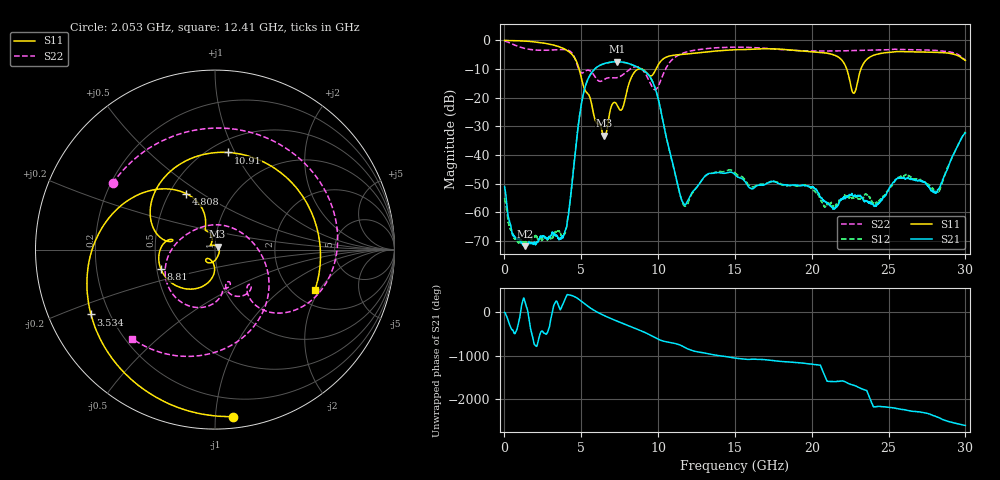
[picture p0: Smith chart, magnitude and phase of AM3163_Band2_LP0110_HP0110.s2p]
!Agilent Technologies,E8364B,MY43040894,A.07.50.67
!Agilent E8364B: A.07.50.67
!Date: Thursday, August 20, 2020 11:12:03
!Correction: S11(Full 2 Port(1,2))
!S21(Full 2 Port(1,2))
!S12(Full 2 Port(1,2))
!S22(Full 2 Port(1,2))
!S2P File: Measurements: S11, S21, S12, S22:
# Hz S  dB  R 50
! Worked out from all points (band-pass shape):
!   3201 points, 10 MHz to 30 GHz, reference 50 ohm
!   highest |S21| = -7.42 dB at 7.348 GHz (marker M1); lowest = -71.7 dB at 1.341 GHz (marker M2)
!   |S21| within 3 dB of the highest: 5.796 GHz to 9.039 GHz (3.244 GHz wide, 43.7 % of centre)
!   lowest |S11| = -33.3 dB at 6.495 GHz (marker M3), VSWR 1.04, Z = 51.4 + j1.67 ohm
!   |S11| at or under -10 dB: 4.86 GHz to 8.714 GHz (3.855 GHz wide, 56.8 % of centre); 8.953 GHz to 9.862 GHz (909.1 MHz wide, 9.66 % of centre); 22.28 GHz to 23.2 GHz (917.5 MHz wide, 4.04 % of centre)
!   |S22| runs from -17.2 to -0.2 dB; largest |S21 - S12| = 0.0047
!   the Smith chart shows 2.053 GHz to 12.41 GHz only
!   S11 on the Smith chart (normalised r, x): 2.053 GHz: 0.07, -1.11; 3.534 GHz: 0.13, -0.24; 4.808 GHz: 0.61, +0.43; 8.81 GHz: 0.53, -0.12; 10.91 GHz: 0.61, +0.94; 12.41 GHz: 2.59, -1.82
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1e7  -0.01 -2.7  -50.94 -9.7  -54.99 -76.7  -0.23 -9.9
6.098e8  -0.08 -24.5  -68.00 -115.6  -69.00 -131.0  -1.50 -81.9
1.340806e9  -0.24 -54.2  -71.75 -133.2  -70.00 -179.4  -2.81 -156.1
2.053069e9  -0.57 -83.9  -70.70 -59.0  -68.19 -64.9  -3.36 147.0
3.533825e9  -2.16 -152.4  -69.25 129.5  -66.59 -24.1  -3.18 43.8
4.05865e9  -3.43 177.1  -64.76 21.8  -64.62 48.4  -3.30 3.1
4.8084e9  -9.08 117.3  -29.48 -60.4  -29.47 -60.9  -9.70 -54.4
5.014581e9  -13.38 106.6  -21.94 -115.8  -21.96 -116.1  -11.34 -47.8
6.495338e9  -33.27 48.3  -8.09 -82.6  -8.10 -82.7  -13.62 -65.8
7.348178e9  -22.69 -133.2  -7.42 148.0  -7.45 147.9  -12.95 -78.6
8.810191e9  -9.89 -160.6  -9.70 -58.4  -9.71 -58.3  -9.51 -139.6
1.000979e10  -8.49 158.6  -20.46 97.2  -20.37 96.6  -15.94 45.9
1.090949e10  -5.25 82.2  -41.99 13.5  -42.20 11.7  -6.73 -58.3
1.167798e10  -4.82 24.6  -56.97 -80.0  -57.59 -76.2  -4.32 -102.1
1.240899e10  -4.43 -22.0  -51.87 178.3  -51.95 -179.8  -3.38 -132.9
1.5005e10  -3.25 -142.2  -46.82 24.2  -46.20 25.0  -2.34 136.0
1.773222e10  -2.99 94.3  -49.60 -43.3  -49.40 -44.8  -3.07 32.2
2.000958e10  -3.94 -26.2  -51.10 -114.5  -51.99 -115.6  -3.68 -49.1
2.27368e10  -18.41 -109.2  -54.33 121.4  -54.94 121.4  -3.53 -126.2
2.500479e10  -4.18 -150.9  -51.99 -23.1  -52.11 -22.0  -3.23 178.1
2.822872e10  -4.17 108.2  -51.90 107.2  -52.84 111.9  -3.54 91.7
3e10  -6.99 43.5  -32.27 -78.6  -31.87 -77.5  -6.82 37.1
